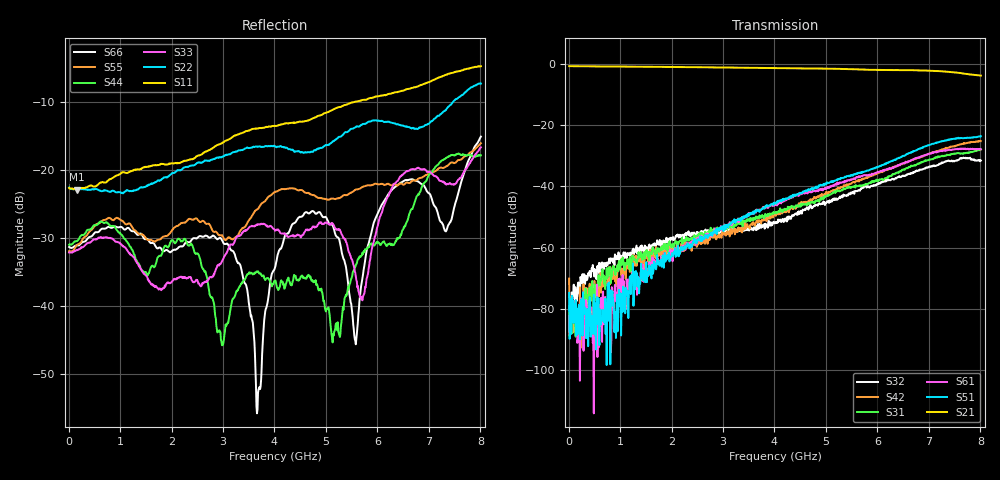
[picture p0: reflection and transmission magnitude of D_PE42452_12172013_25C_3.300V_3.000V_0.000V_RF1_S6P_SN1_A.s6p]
! Device ID: PE42422_06252012
! Dir: z:\David_A\42452\10_28_13_42452_omar_meas\25C\3p300000\RF1
! Serial: 1
! Insertion: A
! Temp: 25C
! VDD: 3.300
! Control_Hi: 3.000
! Control_Lo: 0.000
! Logic State: RF1
! Port 1: RFC
! Port 2: RF1
! Port 3: RF2
! Port 4: RF3
! Port 5: RF4
! Port 6: RF5
! ThroughPath:2-1
! V1 = 3.00
! V2 = 0.00
! V3 = 0.00
! V4 = 0.00
#  Hz  S  RI  R  50
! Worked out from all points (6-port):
!   801 points, 10 MHz to 8.01 GHz, reference 50 ohm
!   strongest paths, dB at 10 MHz, 2.01 GHz, 4.01 GHz, 6.01 GHz, 8.01 GHz:
!     S21: -0.8, -1.0, -1.4, -2.0, -3.9
!     S51: -74.7, -61.8, -45.3, -33.6, -23.6
!     S61: -82.3, -62.3, -46.1, -35.4, -27.9
!     S31: -78.9, -58.8, -48.9, -37.9, -27.9
!     S42: -70.1, -62.4, -49.1, -35.7, -25.2
!     S32: -79.3, -57.1, -52.0, -39.3, -31.6
!   lowest |S11| = -22.9 dB at 160 MHz (marker M1), VSWR 1.15, Z = 57.4 - j1.94 ohm
!   |S11| at or under -10 dB: start of sweep to 5.565 GHz
